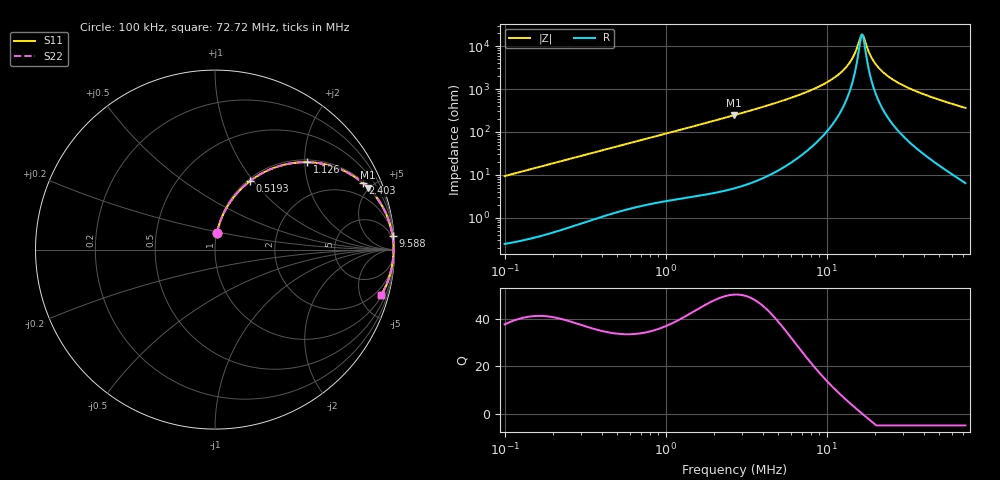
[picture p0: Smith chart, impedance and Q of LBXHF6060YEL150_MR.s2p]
! LBXHF6060YEL150_MR  S-PARAMETER MODEL  ( General Type )
! Model Generated by TAIYO YUDEN Corporation (http://www.ty-top.com)
! Version 1.0
! TAIYO YUDEN Control No. 20211118
! Copyright(c) 2021 TAIYO YUDEN CO.,LTD. All Rights Reserved.
! Product Description (link to TY-COMPAS)
! https://ds.yuden.co.jp/TYCOMPAS/or/detail?pn=LBXHF6060YEL150MMR&u=M
! Products Name : Inductors
! Characteristics :
!  Inductance : 15 uH , SRF(min) : 13 MHz , DC Resistance(max) : 0.105 Ohm
!  Rated Current : Saturation :3100 mA , Temp Rise : 1400 mA
!  Case Size : 6.0 x 6.0 / 0.236 x 0.236 [mm/inch] , Thickness : 4.5 / 0.177 [mm/inch]
!  (Conditions: Temperature = 25 degC , DC Bias Current/Voltage = 0A / 0V)
! External Node Assignments :
!  1  o---GGG---o  2
! GND o---------o GND
! Frequency Range : 0.1MHz  -  72.722828MHz  [ 402 STEP ]
# MHz S RI R 50
! Freq[MHz].  S11 Real  S11 Imag  S21 Real  S21 Imag  S12 Real  S12 Imag  S22 Real  S22 Imag
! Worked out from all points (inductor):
!   401 points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, 100 kHz to 72.72 MHz, reference 50 ohm
!   read as one part in series: L = 15 uH near 103.3 kHz
!   highest Q = 50.5 at 2.653 MHz (marker M1), where L = 14.7 uH
!   self-resonance near 16.51 MHz
!   S11 on the Smith chart (normalised r, x): 100 kHz: 1.00, +0.19; 519.3 kHz: 1.03, +0.96; 1.126 MHz: 1.05, +2.05; 2.403 MHz: 1.09, +4.41; 9.588 MHz: 3, +26; 72.72 MHz: 1.13, -7.27
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0.1  0.0112 0.0929  0.9888 -0.0929  0.9888 -0.0929  0.0112 0.0929
0.30153  0.0791 0.2569  0.9209 -0.2569  0.9209 -0.2569  0.0791 0.2569
0.519299  0.1938 0.3808  0.8062 -0.3808  0.8062 -0.3808  0.1938 0.3808
0.909201  0.4101 0.4782  0.5899 -0.4782  0.5899 -0.4782  0.4101 0.4782
1.126326  0.5121 0.4871  0.4879 -0.4871  0.4879 -0.4871  0.5121 0.4871
2.403013  0.8248 0.3703  0.1752 -0.3703  0.1752 -0.3703  0.8248 0.3703
2.652658  0.852 0.3453  0.148 -0.3453  0.148 -0.3453  0.852 0.3453
2.741508  0.8603 0.3369  0.1397 -0.3369  0.1397 -0.3369  0.8603 0.3369
5.126822  0.9585 0.1869  0.0415 -0.1869  0.0415 -0.1869  0.9585 0.1869
8.131398  0.9846 0.1014  0.0154 -0.1014  0.0154 -0.1014  0.9846 0.1014
9.587536  0.9892 0.0757  0.0108 -0.0757  0.0108 -0.0757  0.9892 0.0757
11.68307  0.9926 0.0472  0.00736 -0.0472  0.00736 -0.0472  0.9926 0.0472
13.32878  0.994 0.0291  0.00605 -0.0291  0.00605 -0.0291  0.994 0.0291
14.71349  0.9945 0.016  0.0055 -0.016  0.0055 -0.016  0.9945 0.016
15.97668  0.9947 0.00511  0.00531 -0.00511  0.00531 -0.00511  0.9947 0.00511
16.51182  0.9947 0.000782  0.0053 -0.000782  0.0053 -0.000782  0.9947 0.000782
17.06488  0.9947 -0.00354  0.00533 0.00354  0.00533 0.00354  0.9947 -0.00354
18.52994  0.9944 -0.0144  0.00555 0.0144  0.00555 0.0144  0.9944 -0.0144
19.79205  0.9941 -0.0231  0.0059 0.0231  0.0059 0.0231  0.9941 -0.0231
24.51857  0.9919 -0.0522  0.00815 0.0522  0.00815 0.0522  0.9919 -0.0522
37.01259  0.9812 -0.1151  0.0188 0.1151  0.0188 0.1151  0.9812 -0.1151
72.72283  0.9257 -0.2535  0.0743 0.2535  0.0743 0.2535  0.9257 -0.2535
